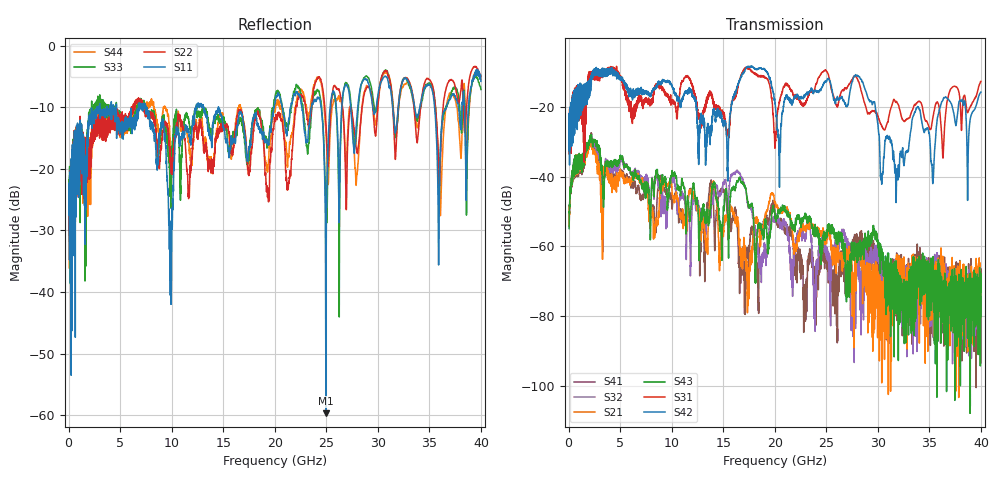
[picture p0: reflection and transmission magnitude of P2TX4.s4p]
!Agilent Technologies,N5245A,MY49151084,A.09.20.08
!Agilent N5245A: A.09.20.08
!Date: Thursday, March 01, 2012 14:38:37
!Correction: S11(Full 4 Port(1,2,3,4))
!S12(Full 4 Port(1,2,3,4))
!S13(Full 4 Port(1,2,3,4))
!S14(Full 4 Port(1,2,3,4))
!S21(Full 4 Port(1,2,3,4))
!S22(Full 4 Port(1,2,3,4))
!S23(Full 4 Port(1,2,3,4))
!S24(Full 4 Port(1,2,3,4))
!S31(Full 4 Port(1,2,3,4))
!S32(Full 4 Port(1,2,3,4))
!S33(Full 4 Port(1,2,3,4))
!S34(Full 4 Port(1,2,3,4))
!S41(Full 4 Port(1,2,3,4))
!S42(Full 4 Port(1,2,3,4))
!S43(Full 4 Port(1,2,3,4))
!S44(Full 4 Port(1,2,3,4))
!S4P File: Measurements: <S11,S12,S13,S14>,
!<S21,S22,S23,S24>,
!<S31,S32,S33,S34>,
!<S41,S42,S43,S44>:
# Hz S  dB  R 50
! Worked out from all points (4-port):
!   3996 points, 50 MHz to 40 GHz, reference 50 ohm
!   strongest paths, dB at 50 MHz, 10.04 GHz, 20.03 GHz, 30.02 GHz, 40 GHz:
!     S42: -24.7, -13.9, -19.1, -25.4, -15.8
!     S31: -24.9, -19.0, -31.1, -22.6, -12.7
!     S43: -54.9, -38.3, -51.3, -59.7, -80.2
!     S21: -53.0, -44.5, -47.2, -70.2, -70.9
!     S32: -52.6, -39.4, -51.5, -60.9, -69.4
!     S41: -52.8, -49.3, -50.6, -62.5, -77.7
!   lowest |S11| = -59.7 dB at 24.96 GHz (marker M1), VSWR 1.00, Z = 49.9 - j0.0862 ohm
!   |S11| at or under -10 dB: start of sweep to 2.777 GHz; 7.468 GHz to 12.39 GHz (4.919 GHz wide, 49.5 % of centre); 14.54 GHz to 19.91 GHz (5.368 GHz wide, 31.2 % of centre)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
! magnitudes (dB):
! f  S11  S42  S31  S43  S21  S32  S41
! 50 MHz  -24.5  -24.7  -24.9  -54.9  -53.0  -52.6  -52.8
! 2.11 GHz  -12.2  -15.7  -11.4  -28.2  -29.8  -29.4  -28.4
! 15.41 GHz  -15.7  -37.4  -28.1  -47.3  -52.2  -47.5  -52.3
! 17.4 GHz  -18.2  -8.5  -9.0  -47.4  -71.6  -48.4  -63.2
! 24.96 GHz  -59.7  -12.7  -9.6  -57.2  -59.0  -61.9  -62.2
! 31.9 GHz  -11.8  -39.2  -19.0  -69.7  -74.3  -66.3  -65.5
! 40 GHz  -5.8  -15.8  -12.7  -80.2  -70.9  -69.4  -77.7
